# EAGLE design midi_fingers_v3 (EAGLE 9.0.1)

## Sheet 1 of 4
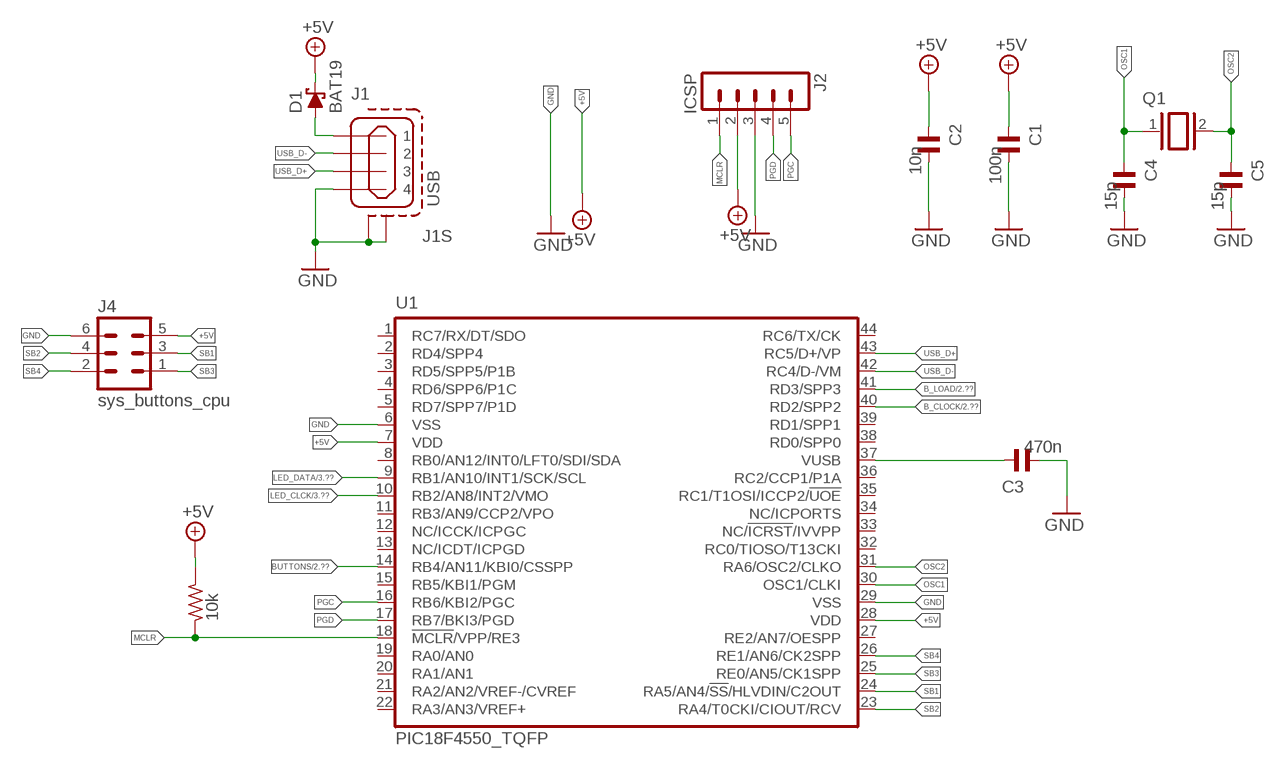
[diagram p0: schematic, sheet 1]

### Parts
C1  100n  C-EUC0603  [C0603]
C2  10n  C-EUC0603  [C0603]
C3  470n  C-EUC0603K  [C0603K]
C4  15p  C-EUC0603  [C0603]
C5  15p  C-EUC0603  [C0603]
D1  BAT19  [DO35-10]
J1  USB  MINI-USB_SHIELD4P-85-32004-00X  [85-32004-00X]
J2  ICSP  MA05-1  [MA05-1]
J4  sys_buttons_cpu  MA03-2  [MA03-2]
Q1  XTAL/S  [QS]
R2  10k  R-EU_M2012  [M2012]
U1  PIC18F4550_TQFP  [TQFP44]

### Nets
+5V: C1.2 C2.2 D1.C J2.2 J4.5 R2.1 U1.7(VDD) U1.28(VDD) ; also sheet 2,3,4
+5V__: D1.A J1.1
B_CLOCK: U1.40(RD2/SPP2) ; also sheet 2
B_LOAD: U1.41(RD3/SPP3) ; also sheet 2
BUTTONS: U1.14(RB4/AN11/KBI0/CSSPP) ; also sheet 2
GND: C1.1 C2.1 C3.1 C4.1 C5.1 J1.4 J1.M1(S1) J1.M2(S2) J2.3 J4.6 U1.6(VSS) U1.29(VSS) ; also sheet 2,3,4
LED_CLCK: U1.10(RB2/AN8/INT2/VMO) ; also sheet 3
LED_DATA: U1.9(RB1/AN10/INT1/SCK/SCL) ; also sheet 3
MCLR: J2.1 R2.2 U1.18(!MCLR!/VPP/RE3)
N$5: C3.2 U1.37(VUSB)
OSC1: C4.2 Q1.1 U1.30(OSC1/CLKI)
OSC2: C5.2 Q1.2 U1.31(RA6/OSC2/CLKO)
PGC: J2.5 U1.16(RB6/KBI2/PGC)
PGD: J2.4 U1.17(RB7/BKI3/PGD)
SB1: J4.3 U1.24(RA5/AN4/!SS!/HLVDIN/C2OUT)
SB2: J4.4 U1.23(RA4/T0CKI/CIOUT/RCV)
SB3: J4.1 U1.25(RE0/AN5/CK1SPP)
SB4: J4.2 U1.26(RE1/AN6/CK2SPP)
USB_D+: J1.3 U1.43(RC5/D+/VP)
USB_D-: J1.2 U1.42(RC4/D-/VM)
Unconnected: U1.1(RC7/RX/DT/SDO) U1.2(RD4/SPP4) U1.3(RD5/SPP5/P1B) U1.4(RD6/SPP6/P1C) U1.5(RD7/SPP7/P1D) U1.8(RB0/AN12/INT0/LFT0/SDI/SDA) U1.11(RB3/AN9/CCP2/VPO) U1.12(NC/ICCK/ICPGC) U1.13(NC/ICDT/ICPGD) U1.15(RB5/KBI1/PGM) U1.19(RA0/AN0) U1.20(RA1/AN1) U1.21(RA2/AN2/VREF-/CVREF) U1.22(RA3/AN3/VREF+) U1.27(RE2/AN7/OESPP) U1.32(RC0/TIOSO/T13CKI) U1.33(NC/!ICRST!/IVVPP) U1.34(NC/ICPORTS) U1.35(RC1/T1OSI/ICCP2/!UOE) U1.36(RC2/CCP1/P1A) U1.38(RD0/SPP0) U1.39(RD1/SPP1) U1.44(RC6/TX/CK)

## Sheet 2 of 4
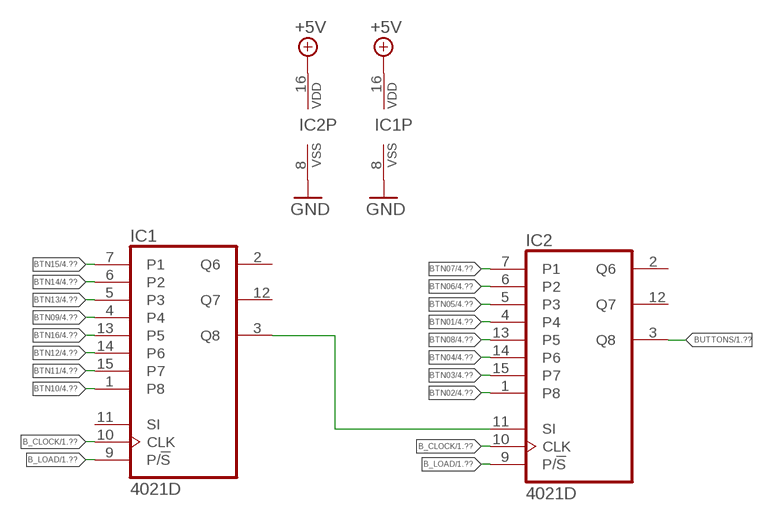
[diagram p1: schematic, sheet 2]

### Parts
IC1  4021D  [SO16]
IC2  4021D  [SO16]

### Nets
+5V: IC1.16(VDD) IC2.16(VDD) ; also sheet 1,3,4
B_CLOCK: IC1.10(CLK) IC2.10(CLK) ; also sheet 1
B_LOAD: IC1.9(P/!S) IC2.9(P/!S) ; also sheet 1
BTN01: IC2.4 ; also sheet 4
BTN02: IC2.1(P8) ; also sheet 4
BTN03: IC2.15(P7) ; also sheet 4
BTN04: IC2.14(P6) ; also sheet 4
BTN05: IC2.5(P3) ; also sheet 4
BTN06: IC2.6(P2) ; also sheet 4
BTN07: IC2.7(P1) ; also sheet 4
BTN08: IC2.13(P5) ; also sheet 4
BTN09: IC1.4 ; also sheet 4
BTN10: IC1.1(P8) ; also sheet 4
BTN11: IC1.15(P7) ; also sheet 4
BTN12: IC1.14(P6) ; also sheet 4
BTN13: IC1.5(P3) ; also sheet 4
BTN14: IC1.6(P2) ; also sheet 4
BTN15: IC1.7(P1) ; also sheet 4
BTN16: IC1.13(P5) ; also sheet 4
BTN_SERIAL: IC1.3(Q8) IC2.11(SI)
BUTTONS: IC2.3(Q8) ; also sheet 1
GND: IC1.8(VSS) IC2.8(VSS) ; also sheet 1,3,4
Unconnected: IC1.2(Q6) IC1.11(SI) IC1.12(Q7) IC2.2(Q6) IC2.12(Q7)

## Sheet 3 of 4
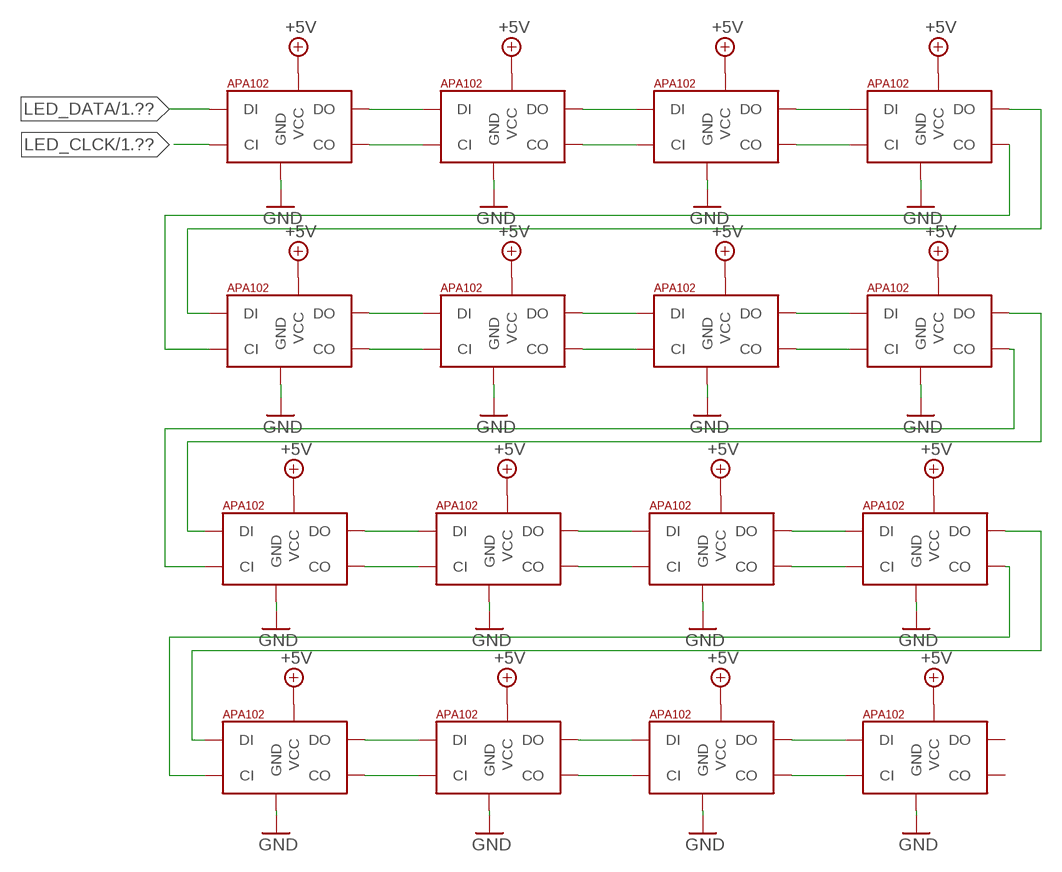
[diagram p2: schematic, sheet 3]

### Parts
LED1  APA1025050  [APA102_5050]
LED2  APA1025050  [APA102_5050]
LED3  APA1025050  [APA102_5050]
LED4  APA1025050  [APA102_5050]
LED5  APA1025050  [APA102_5050]
LED6  APA1025050  [APA102_5050]
LED7  APA1025050  [APA102_5050]
LED8  APA1025050  [APA102_5050]
LED9  APA1025050  [APA102_5050]
LED10  APA1025050  [APA102_5050]
LED11  APA1025050  [APA102_5050]
LED12  APA1025050  [APA102_5050]
LED13  APA1025050  [APA102_5050]
LED14  APA1025050  [APA102_5050]
LED15  APA1025050  [APA102_5050]
LED16  APA1025050  [APA102_5050]

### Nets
+5V: LED1.1(VCC) LED2.1(VCC) LED3.1(VCC) LED4.1(VCC) LED5.1(VCC) LED6.1(VCC) LED7.1(VCC) LED8.1(VCC) LED9.1(VCC) LED10.1(VCC) LED11.1(VCC) LED12.1(VCC) LED13.1(VCC) LED14.1(VCC) LED15.1(VCC) LED16.1(VCC) ; also sheet 1,2,4
GND: LED1.6(GND) LED2.6(GND) LED3.6(GND) LED4.6(GND) LED5.6(GND) LED6.6(GND) LED7.6(GND) LED8.6(GND) LED9.6(GND) LED10.6(GND) LED11.6(GND) LED12.6(GND) LED13.6(GND) LED14.6(GND) LED15.6(GND) LED16.6(GND) ; also sheet 1,2,4
LED_CLCK: LED1.5(CI) ; also sheet 1
LED_DATA: LED1.4(DI) ; also sheet 1
N$1: LED1.3(DO) LED2.4(DI)
N$2: LED2.3(DO) LED3.4(DI)
N$3: LED3.3(DO) LED4.4(DI)
N$4: LED5.3(DO) LED6.4(DI)
N$6: LED6.3(DO) LED7.4(DI)
N$7: LED7.3(DO) LED8.4(DI)
N$8: LED9.3(DO) LED10.4(DI)
N$9: LED10.3(DO) LED11.4(DI)
N$10: LED11.3(DO) LED12.4(DI)
N$11: LED13.3(DO) LED14.4(DI)
N$12: LED14.3(DO) LED15.4(DI)
N$13: LED15.3(DO) LED16.4(DI)
N$14: LED8.3(DO) LED9.4(DI)
N$15: LED12.3(DO) LED13.4(DI)
N$16: LED1.2(CO) LED2.5(CI)
N$17: LED2.2(CO) LED3.5(CI)
N$18: LED3.2(CO) LED4.5(CI)
N$19: LED4.3(DO) LED5.4(DI)
N$20: LED4.2(CO) LED5.5(CI)
N$21: LED5.2(CO) LED6.5(CI)
N$22: LED6.2(CO) LED7.5(CI)
N$23: LED7.2(CO) LED8.5(CI)
N$24: LED8.2(CO) LED9.5(CI)
N$25: LED9.2(CO) LED10.5(CI)
N$26: LED10.2(CO) LED11.5(CI)
N$27: LED11.2(CO) LED12.5(CI)
N$28: LED12.2(CO) LED13.5(CI)
N$30: LED13.2(CO) LED14.5(CI)
N$31: LED14.2(CO) LED15.5(CI)
N$32: LED15.2(CO) LED16.5(CI)
Unconnected: LED16.2(CO) LED16.3(DO)

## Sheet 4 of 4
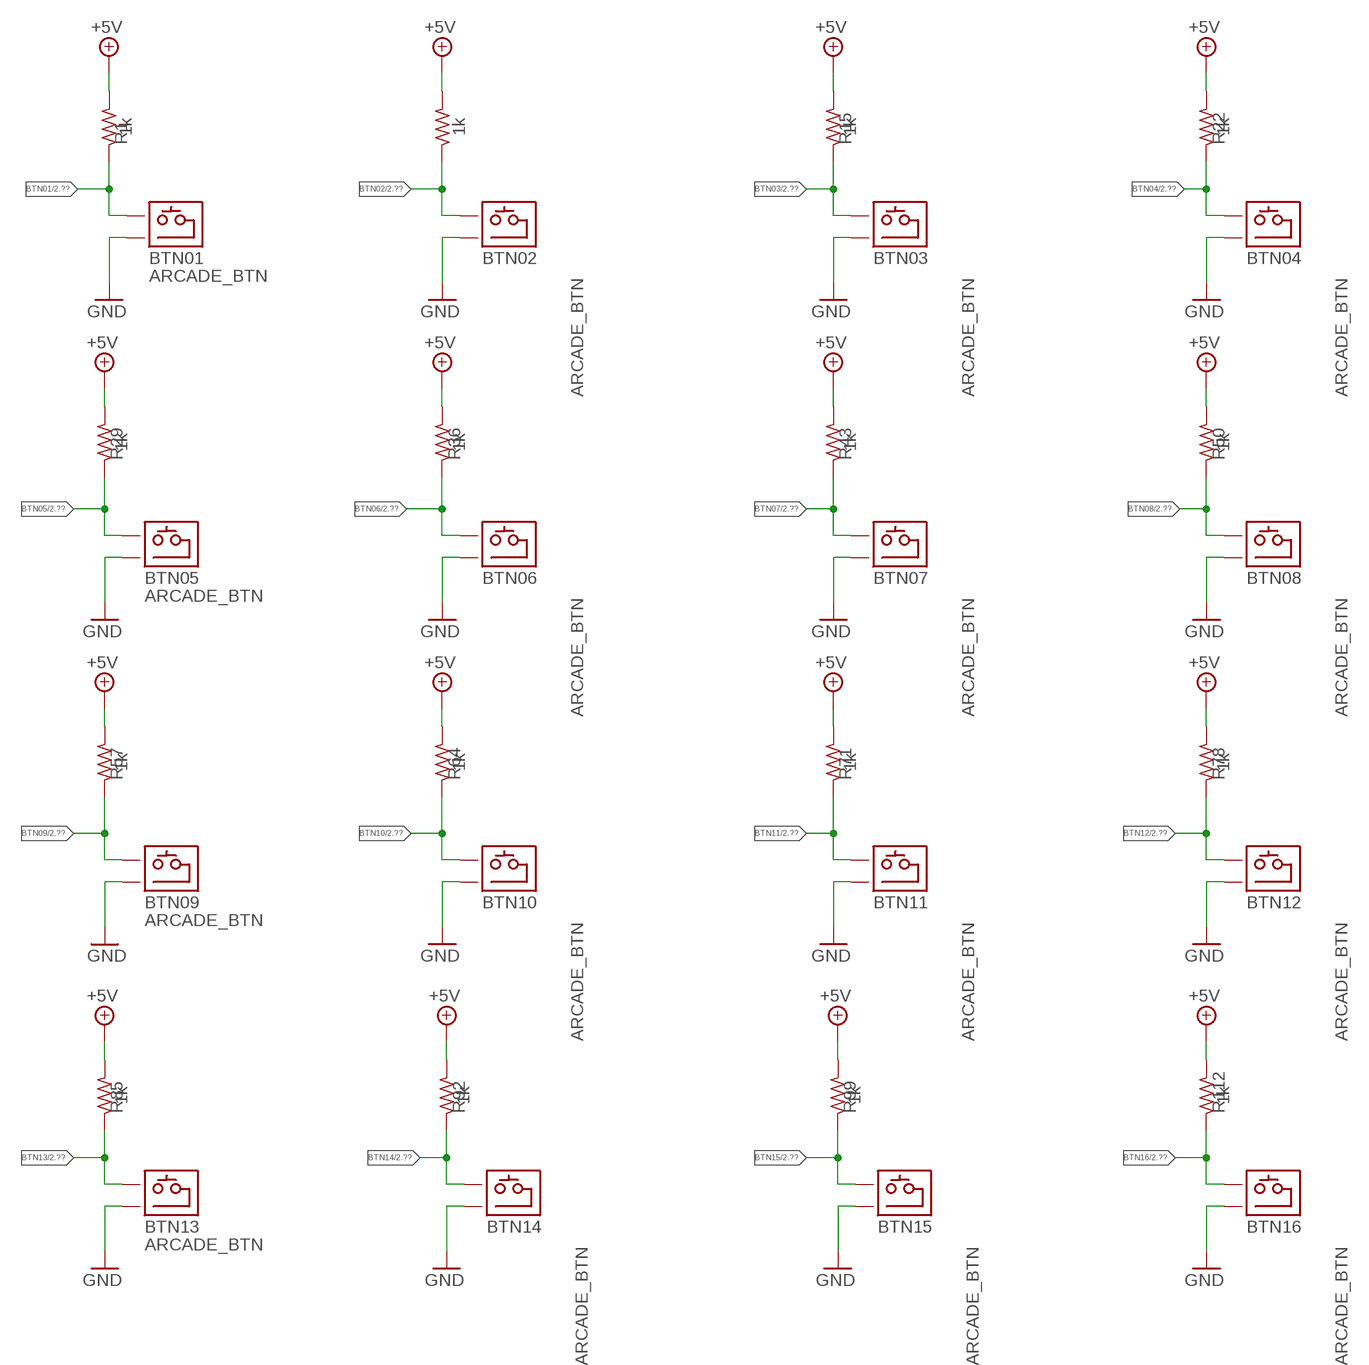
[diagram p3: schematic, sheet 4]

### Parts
BTN01  ARCADE_BTN  [ARCADE_BTN_ALONE]
BTN02  ARCADE_BTN  [ARCADE_BTN_ALONE]
BTN03  ARCADE_BTN  [ARCADE_BTN_ALONE]
BTN04  ARCADE_BTN  [ARCADE_BTN_ALONE]
BTN05  ARCADE_BTN  [ARCADE_BTN_ALONE]
BTN06  ARCADE_BTN  [ARCADE_BTN_ALONE]
BTN07  ARCADE_BTN  [ARCADE_BTN_ALONE]
BTN08  ARCADE_BTN  [ARCADE_BTN_ALONE]
BTN09  ARCADE_BTN  [ARCADE_BTN_ALONE]
BTN10  ARCADE_BTN  [ARCADE_BTN_ALONE]
BTN11  ARCADE_BTN  [ARCADE_BTN_ALONE]
BTN12  ARCADE_BTN  [ARCADE_BTN_ALONE]
BTN13  ARCADE_BTN  [ARCADE_BTN_ALONE]
BTN14  ARCADE_BTN  [ARCADE_BTN_ALONE]
BTN15  ARCADE_BTN  [ARCADE_BTN_ALONE]
BTN16  ARCADE_BTN  [ARCADE_BTN_ALONE]
R1  1k  R-EU_M2012  [M2012]
R8  1k  R-EU_M2012  [M2012]
R15  1k  R-EU_M2012  [M2012]
R22  1k  R-EU_M2012  [M2012]
R29  1k  R-EU_M2012  [M2012]
R36  1k  R-EU_M2012  [M2012]
R43  1k  R-EU_M2012  [M2012]
R50  1k  R-EU_M2012  [M2012]
R57  1k  R-EU_M2012  [M2012]
R64  1k  R-EU_M2012  [M2012]
R71  1k  R-EU_M2012  [M2012]
R78  1k  R-EU_M2012  [M2012]
R85  1k  R-EU_M2012  [M2012]
R92  1k  R-EU_M2012  [M2012]
R99  1k  R-EU_M2012  [M2012]
R112  1k  R-EU_M2012  [M2012]

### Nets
+5V: R1.1 R8.1 R15.1 R22.1 R29.1 R36.1 R43.1 R50.1 R57.1 R64.1 R71.1 R78.1 R85.1 R92.1 R99.1 R112.1 ; also sheet 1,2,3
BTN01: BTN01.1(B1) R1.2 ; also sheet 2
BTN02: BTN02.1(B1) R8.2 ; also sheet 2
BTN03: BTN03.1(B1) R15.2 ; also sheet 2
BTN04: BTN04.1(B1) R22.2 ; also sheet 2
BTN05: BTN05.1(B1) R29.2 ; also sheet 2
BTN06: BTN06.1(B1) R36.2 ; also sheet 2
BTN07: BTN07.1(B1) R43.2 ; also sheet 2
BTN08: BTN08.1(B1) R50.2 ; also sheet 2
BTN09: BTN09.1(B1) R57.2 ; also sheet 2
BTN10: BTN10.1(B1) R64.2 ; also sheet 2
BTN11: BTN11.1(B1) R71.2 ; also sheet 2
BTN12: BTN12.1(B1) R78.2 ; also sheet 2
BTN13: BTN13.1(B1) R85.2 ; also sheet 2
BTN14: BTN14.1(B1) R92.2 ; also sheet 2
BTN15: BTN15.1(B1) R99.2 ; also sheet 2
BTN16: BTN16.1(B1) R112.2 ; also sheet 2
GND: BTN01.2(B2) BTN02.2(B2) BTN03.2(B2) BTN04.2(B2) BTN05.2(B2) BTN06.2(B2) BTN07.2(B2) BTN08.2(B2) BTN09.2(B2) BTN10.2(B2) BTN11.2(B2) BTN12.2(B2) BTN13.2(B2) BTN14.2(B2) BTN15.2(B2) BTN16.2(B2) ; also sheet 1,2,3

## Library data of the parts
BTN01-BTN09 BTN10-BTN16 = arcade-button:ARCADE_BTN
C1-C5 = rcl:C-EU: CAPACITOR, European symbol
D1 = diode:BAT19: DIODE
IC1 IC2 = 40xx:4021: 8-bit static SHIFT REGISTER
J1 = con-cypressindustries:MINI-USB_SHIELD4P-: MINI USB 4 Pol. Source: www.cypressindustries.com
J2 = con-lstb:MA05-1: PIN HEADER; OC_FARNELL: unknown; OC_NEWARK: unknown
J4 = con-lstb:MA03-2: PIN HEADER
LED1-LED16 = jos-ph:APA102: APA102C 5050 RGB LED -- Adafruit DotStar Single LED Pixel Product Page: https://www.adafruit.com/products/2343 Datasheet: https://cdn-shop.adafruit.com/product-files/2343/APA102C.pdf
Q1 = special:XTAL/S: CRYSTAL
R1 R2 R8 R15 R22 R29 R36 R43 R50 R57 R64 R71 R78 R85 R92 R99 R112 = rcl:R-EU_: RESISTOR, European symbol
U1 = microchip:PIC18F4*_TQFP: USB Microcontrollers with nanoWatt Technology High-Performance, Enhanced Flash, 28/40/44-Pin, Source: http://ww1.microchip.com/downloads/en/devicedoc/39632c.pdf

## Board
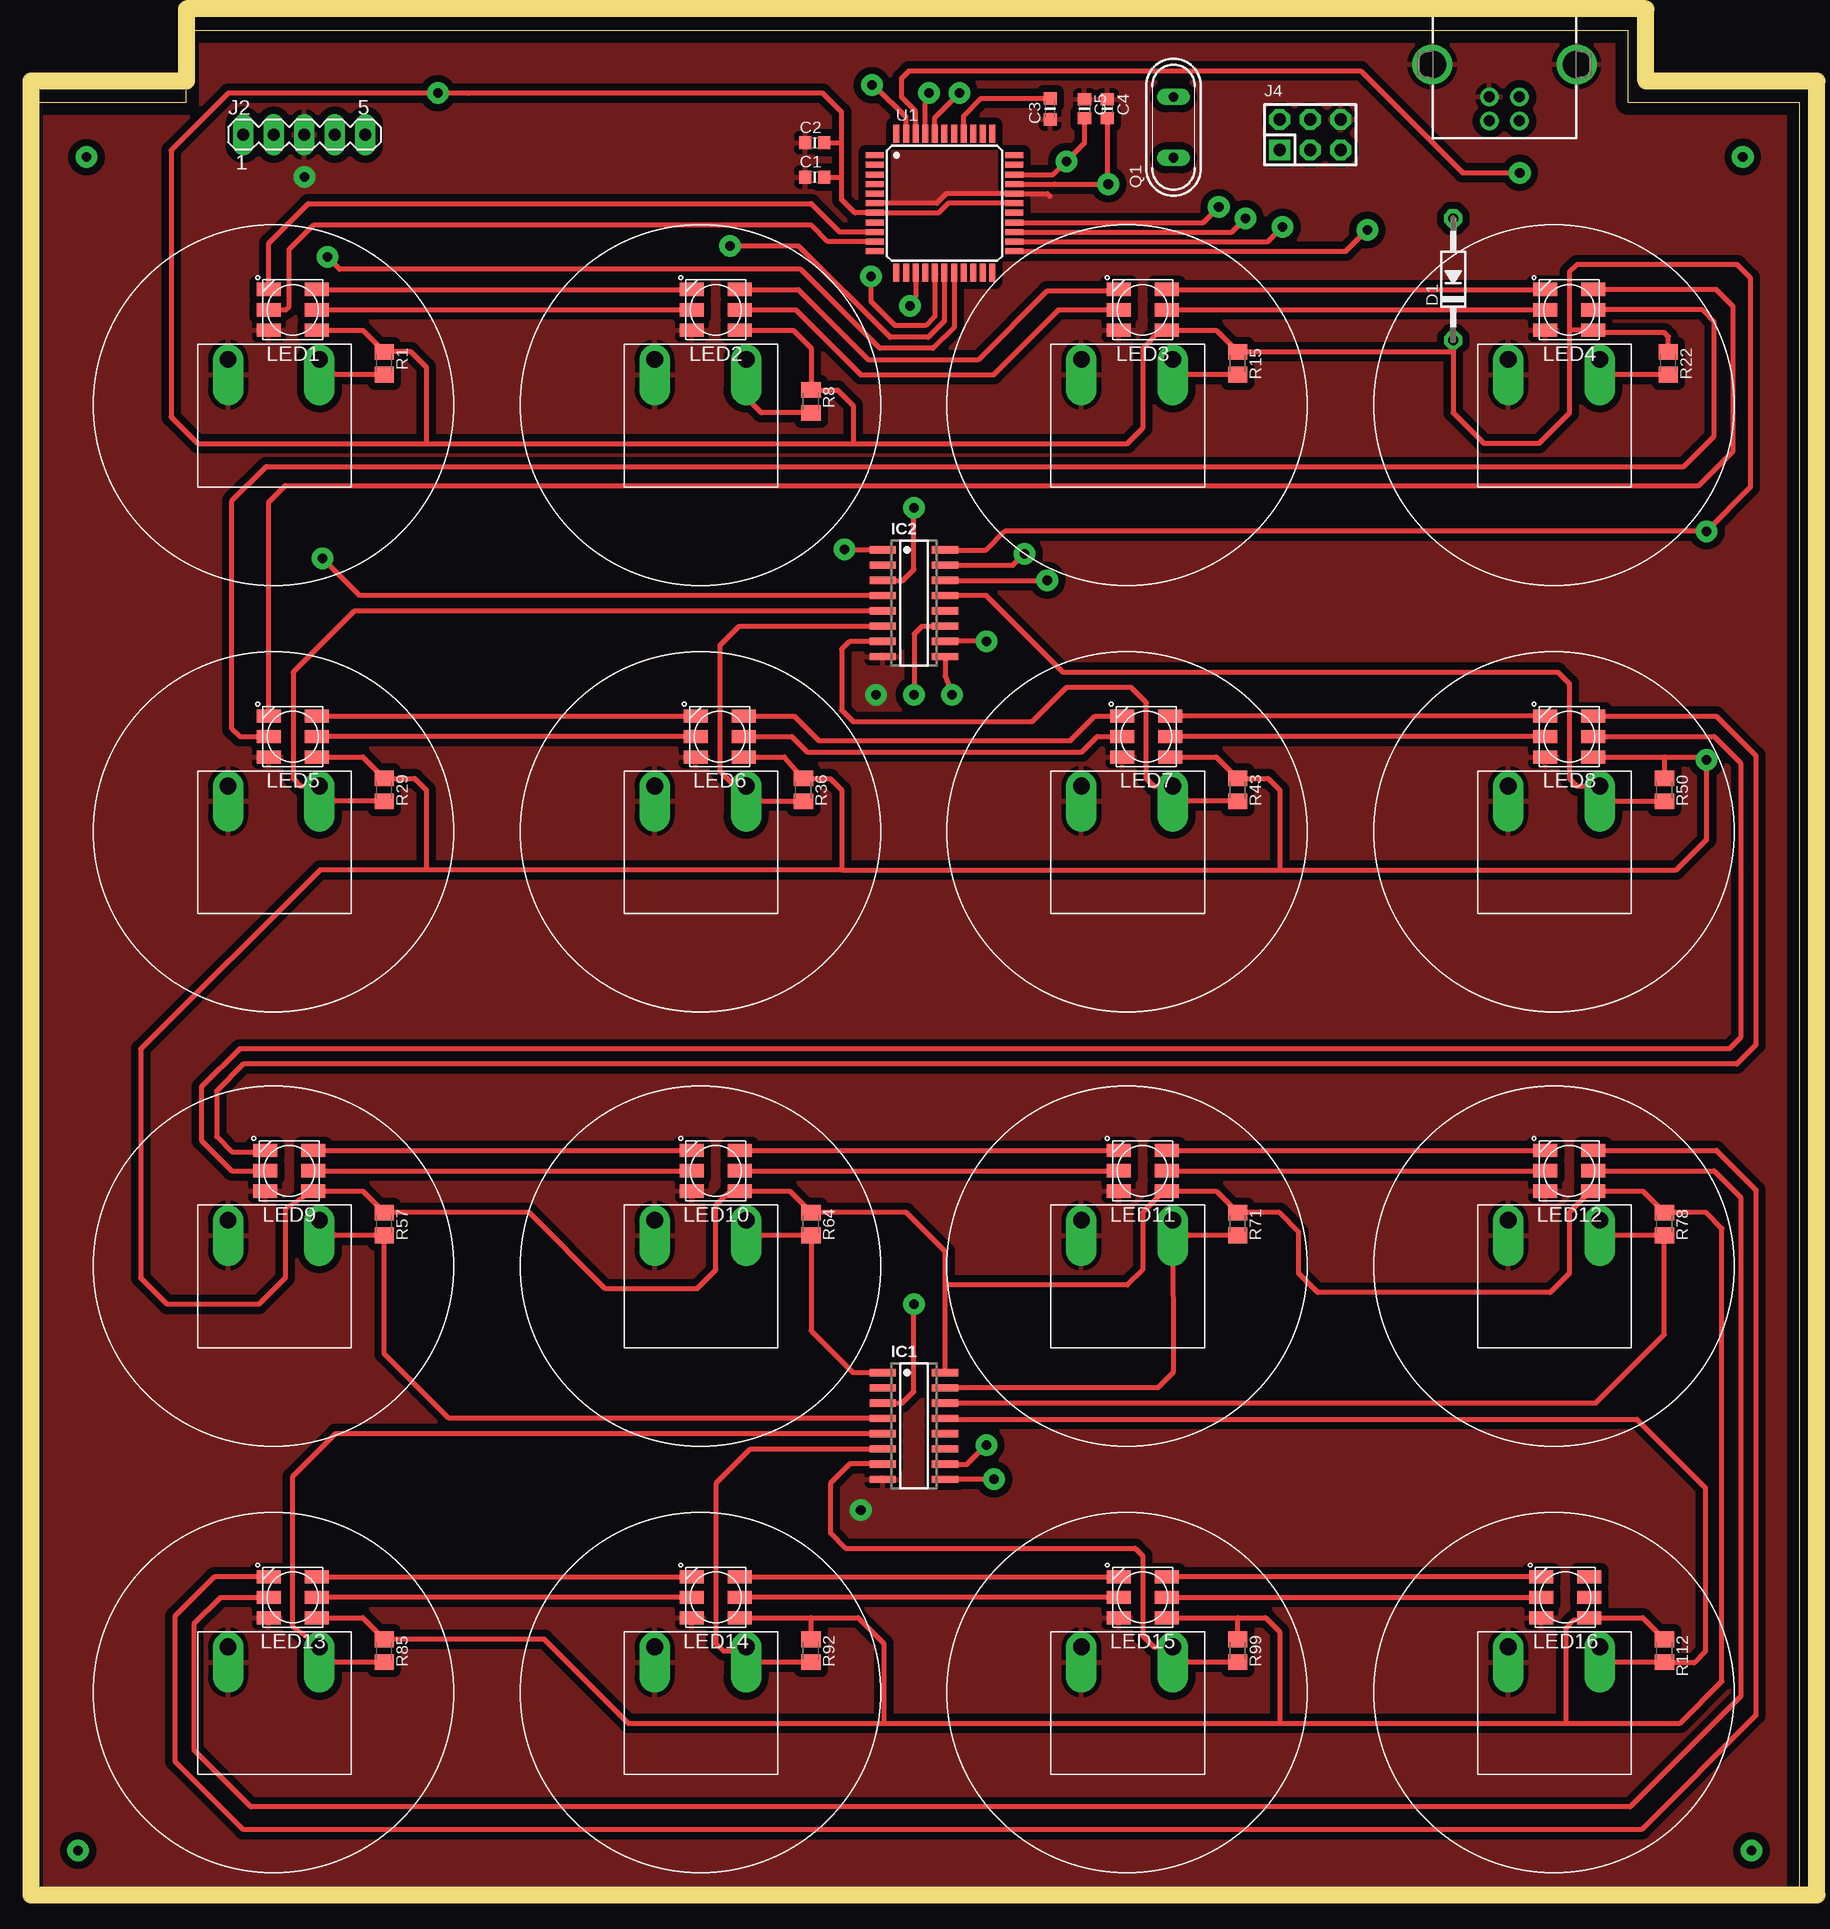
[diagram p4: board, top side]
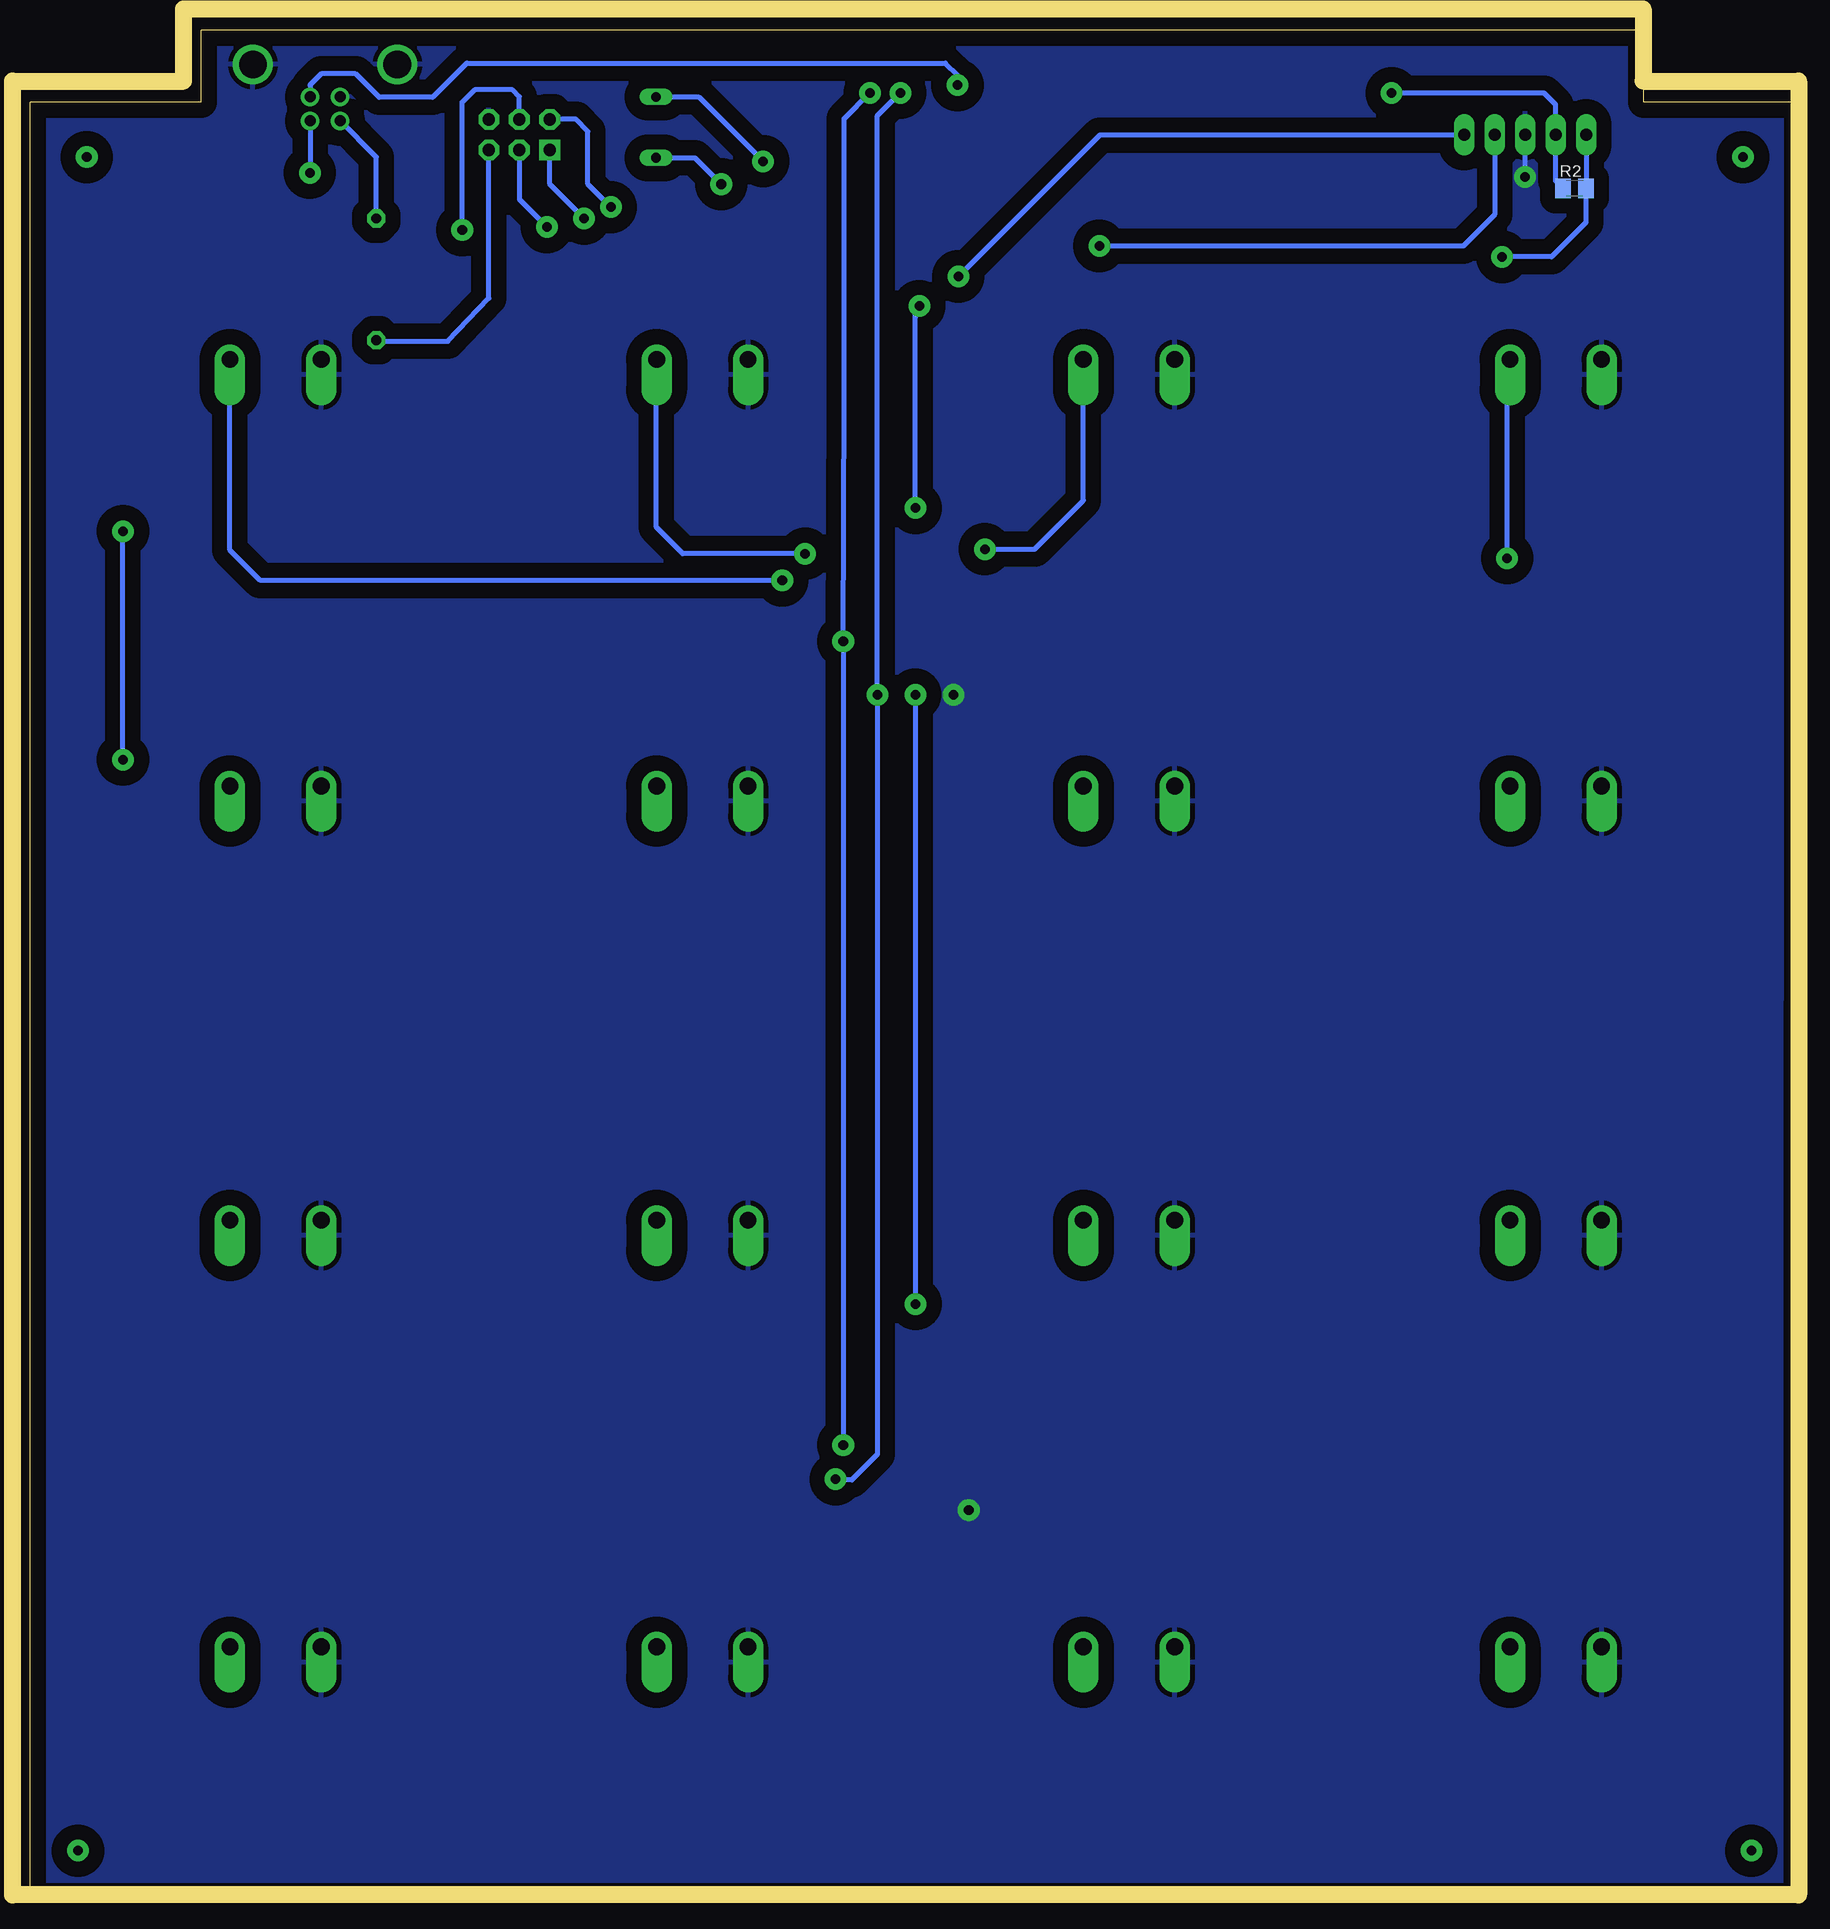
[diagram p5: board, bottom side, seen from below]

Size 147.46 x 155.76 mm. Coordinates in mm from the lower left corner, seen from the top.
Outline: 0.01,0 147.46,0 147.46,149.76 133.19,149.76 133.19,155.76 13,155.76 13,149.76 0,149.76 0.01,0
Copper layers (1*16): Top 0.035mm / dielectric 1.5mm / Bottom 0.035mm
Design rules "default *": minimum track width 10mil, minimum drill 0.6mm, track to track 8mil, track to pad 8mil, pad to pad 8mil, via to via 8mil, smd to smd 8mil, copper to edge 40mil, drill to drill 6mil, minimum pad ring 0mil, minimum via ring 8mil, stop-mask expansion 4mil, vias tented up to drill 0mil, thermal gap 16mil
Milling: 8 lines

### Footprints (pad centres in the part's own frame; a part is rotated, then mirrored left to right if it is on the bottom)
ARCADE_BTN_ALONE = drill 1.4 pad 2.54 offset: 1 3.81,3.81; 2 -3.81,3.81
C0603 = smd 1 x 1.1: 1 -0.794,0; 2 0.794,0
C0603K = smd 1.05 x 1.08: 1 -0.875,0; 2 0.875,0
DO35-10 = drill 0.813 pad 1.524 octagon: A 5.08,0; C -5.08,0
SO16 = smd 0.6 x 2.2: 1 -4.445,-2.6; 2 -3.175,-2.6; 3 -1.905,-2.6; 4 -0.635,-2.6; 5 0.635,-2.6; 6 1.905,-2.6; 7 3.175,-2.6; 8 4.445,-2.6; 9 4.445,2.6; 10 3.175,2.6; 11 1.905,2.6; 12 0.635,2.6; 13 -0.635,2.6; 14 -1.905,2.6; 15 -3.175,2.6; 16 -4.445,2.6
85-32004-00X = drill 0.92 pad 1.27: 1 4.71,-1.25; 2 4.71,1.25; 3 2.71,1.25; 4 2.71,-1.25 | drill 2.3 pad 3: M1 0,6.02; M2 0,-6.02
MA05-1 = drill 1.016 long: 1 -5.08,0; 2 -2.54,0; 3 0,0; 4 2.54,0; 5 5.08,0
MA03-2 = drill 1.016 square: 1 -2.54,-1.27 | drill 1.016 octagon: 2 -2.54,1.27; 3 0,-1.27; 4 0,1.27; 5 2.54,-1.27; 6 2.54,1.27
APA102_5050 = smd 2 x 1.1: 1 2,-1.7; 2 2,0; 3 2,1.7; 4 -2,1.7; 5 -2,0; 6 -2,-1.7
QS = drill 0.8 long: 1 -2.54,0; 2 2.54,0
M2012 = smd 1.3 x 1.6: 1 -0.95,0; 2 0.95,0
TQFP44 = smd 1.5 x 0.5: 1 -5.8,4; 2 -5.8,3.2; 3 -5.8,2.4; 4 -5.8,1.6; 5 -5.8,0.8; 6 -5.8,0; 7 -5.8,-0.8; 8 -5.8,-1.6; 9 -5.8,-2.4; 10 -5.8,-3.2; 11 -5.8,-4; 23 5.8,-4; 24 5.8,-3.2; 25 5.8,-2.4; 26 5.8,-1.6; 27 5.8,-0.8; 28 5.8,0; 29 5.8,0.8; 30 5.8,1.6; 31 5.8,2.4; 32 5.8,3.2; 33 5.8,4 | smd 0.5 x 1.5: 12 -4,-5.8; 13 -3.2,-5.8; 14 -2.4,-5.8; 15 -1.6,-5.8; 16 -0.8,-5.8; 17 0,-5.8; 18 0.8,-5.8; 19 1.6,-5.8; 20 2.4,-5.8; 21 3.2,-5.8; 22 4,-5.8; 34 4,5.8; 35 3.2,5.8; 36 2.4,5.8; 37 1.6,5.8; 38 0.8,5.8; 39 0,5.8; 40 -0.8,5.8; 41 -1.6,5.8; 42 -2.4,5.8; 43 -3.2,5.8; 44 -4,5.8

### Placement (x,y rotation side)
BTN01  20.31,124.49 0 top
BTN02  55.87,124.49 0 top
BTN03  91.43,124.49 0 top
BTN04  126.99,124.49 0 top
BTN05  20.31,88.93 0 top
BTN06  55.87,88.93 0 top
BTN07  91.43,88.93 0 top
BTN08  126.99,88.93 0 top
BTN09  20.31,52.73 0 top
BTN10  55.87,52.73 0 top
BTN11  91.43,52.73 0 top
BTN12  126.99,52.73 0 top
BTN13  20.31,17.17 0 top
BTN14  55.87,17.17 0 top
BTN15  91.43,17.17 0 top
BTN16  126.99,17.17 0 top
C1  65.39,143.5 0 top
C2  65.39,146.35 0 top
C3  85.01,149.19 90 top
C4  89.78,149.19 270 top
C5  87.87,149.19 270 top
D1  118.6,134.97 90 top
IC1  73.66,39.4 270 top
IC2  73.66,107.98 270 top
J1  122.87,152.89 270 top
J2  22.86,147.03 0 top
J4  106.68,147.03 0 top
LED1  21.91,132.43 0 top
LED2  57.15,132.43 0 top
LED3  92.71,132.43 0 top
LED4  128.27,132.43 0 top
LED5  21.91,96.86 0 top
LED6  57.47,96.86 0 top
LED7  93.03,96.86 0 top
LED8  128.27,96.86 0 top
LED9  21.59,60.67 0 top
LED10  57.15,60.67 0 top
LED11  92.71,60.67 0 top
LED12  128.27,60.67 0 top
LED13  21.91,25.11 0 top
LED14  57.15,25.11 0 top
LED15  92.71,25.11 0 top
LED16  127.95,25.11 0 top
Q1  95.29,147.65 90 top
R1  29.53,127.98 270 top
R2  18.75,142.56 0 bottom
R8  65.09,124.81 270 top
R15  100.65,127.98 270 top
R22  136.52,127.98 270 top
R29  29.53,92.42 270 top
R36  64.45,92.42 270 top
R43  100.65,92.42 270 top
R50  136.21,92.42 270 top
R57  29.53,56.23 270 top
R64  65.09,56.23 270 top
R71  100.65,56.23 270 top
R78  136.21,56.23 270 top
R85  29.53,20.66 270 top
R92  65.09,20.66 270 top
R99  100.65,20.66 270 top
R112  136.21,20.66 270 top
U1  76.2,141.31 0 top

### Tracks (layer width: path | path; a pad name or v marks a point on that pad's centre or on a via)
+5V  (via drill 0.8 pad 1.8)
  Top 0.406: R22.1 136.52,130.2 136.21,130.52 130.48,130.52 LED4.1 | R15.1 | R15.1 98.85,130.72 LED3.1 94.18,130.72 92.71,129.25 92.71,122.57 92.72,122.56 91.45,121.28 68.59,121.28 | LED1.1 27.73,130.72 R1.1 | LED5.1 27.73,95.17 R29.1 32.05,93.37 33.03,92.39 33.03,85.75 | LED6.1 62.86,95.17 R36.1 64.48,93.34 66.69,93.34 67.64,92.39 67.64,85.75 | 76.26,51.4 IC1.16 76.33,43.77 | 76.26,51.4 76.26,53.94 73.03,57.18 R64.1 63.29,58.97 LED10.1 | LED10.1 59.15,58.86 | 100.65,23.41 LED15.1 94.17,23.41 | R99.1 100.65,23.41 | LED13.1 27.73,23.41 R85.1 42.86,21.62 49.85,14.63 71.13,14.63 | LED16.1 134.41,23.41 R112.1 | LED16.1 129.74,23.41 | R1.1 | LED7.1 94.82,95.17 | U1.28 76.52,141.31 75.72,140.51 U1.7 68.73,140.51 67.64,141.6 67.64,143.51 | LED14.1 65.09,23.41 | 65.09,23.41 69.01,23.41 71.13,21.29 71.13,14.63 | R92.1 65.09,23.41 | 76.26,51.4 76.51,51.15 91.44,51.15 92.71,52.41 92.71,57.18 94.5,58.97 LED11.1 98.85,58.97 R71.1 104.14,57.18 105.73,55.59 105.73,52.1 107.31,50.51 126.68,50.51 128.27,52.1 128.27,57.18 129.95,58.86 LED12.1 134.41,58.97 R78.1 139.69,57.17 140.98,55.88 140.98,18.1 137.52,14.63 127.97,14.63 | IC2.16 79.68,112.42 81.24,113.98 v139.71,113.98 143.36,117.63 143.36,135.1 142.25,136.21 128.92,136.21 128.28,135.57 128.28,130.81 | 129.73,130.72 LED4.1 | R15.1 118.59,128.93 D1.C 118.6,123.85 121.17,121.28 125.74,121.28 128.28,123.83 128.28,130.81 | LED16.1 129.91,23.45 | LED4.1 128.37,130.72 128.28,130.81 | LED7.1 94.94,95.25 | LED10.1 58.11,58.74 57.16,57.78 57.15,52.41 55.56,50.83 47.94,50.83 41.59,57.18 R57.1 27.73,58.97 LED9.1 21.29,57.47 21.29,51.75 19.06,49.53 11.44,49.53 9.22,51.75 9.22,70.8 24.17,85.75 33.03,85.75
  Top 0.406: LED16.1 129.72,23.18 128.6,23.18 127.97,22.54 127.97,14.63 | 71.13,14.63 104.15,14.63 | 104.15,14.63 127.97,14.63 | 100.65,23.41 102.97,23.41 104.15,22.23 104.15,14.63 | LED8.1 136.22,95.17 | 136.22,95.17 139.48,95.17 v139.71,94.93 139.71,88.27 137.2,85.75 104.15,85.75 | R50.1 136.22,93.38 136.22,95.17 | R43.1 100.66,93.38 | 67.64,85.75 104.15,85.75 | 67.64,143.51 67.64,147 | 67.64,147 67.64,148.91 66.05,150.5 36.53,150.5 | R1.1 31.74,128.93 33.03,127.64 33.03,121.28 | 36.53,150.5 v33.98,150.5 33.67,150.5 | 33.67,150.5 16.52,150.5 11.76,145.73 11.76,123.51 13.98,121.28 33.03,121.28 | J2.2 20.33,147.04 | 58.67,130.72 LED2.1 63.61,130.72 65.09,129.25 R8.1 67.3,125.75 68.59,124.46 68.59,121.28 | 67.64,85.75 33.03,85.75 | LED7.1 98.85,95.17 R43.1 | R43.1 103.17,93.37 104.15,92.39 104.15,85.75 | 33.03,121.28 68.59,121.28 | 33.68,150.48 33.67,150.5 | 36.54,150.48 36.53,150.5 | C2.2 67.63,146.35 67.64,147 | C1.2 67.63,143.5 67.64,143.51
  Bottom 0.406: D1.C 118.52,129.82 112.64,129.82 109.22,133.39 J4.5 | v139.71,94.93 v139.71,113.98 | v33.98,150.5 21.29,150.5 20.32,149.53 J2.2 20.32,143.18 R2.1
+5V__
  Bottom 0.406: D1.A 118.6,145.16 J1.1
B_CLOCK  (via drill 0.8 pad 1.8)
  Top 0.406: U1.40 75.4,148.45 v77.47,150.52 | v79.69,37.81 78.04,36.16 76.44,36.16 IC1.10 | v79.69,104.8 IC2.10
  Bottom 0.406: v79.69,37.81 v79.69,104.8 79.62,125.06 79.62,148.38 v77.47,150.52
B_LOAD  (via drill 0.8 pad 1.8)
  Top 0.406: IC2.9 76.26,101.89 v76.84,100.36 | v80.33,34.95 IC1.9 | U1.41 74.6,150.19 v74.93,150.52
  Bottom 0.406: v80.33,34.95 80.26,34.88 78.98,34.88 76.84,37.03 v76.84,100.36 76.84,148.62 v74.93,150.52
BTN01  (via drill 0.8 pad 1.8)
  Top 0.406: IC2.4 27.48,108.61 v24.37,111.72 | R1.2 25.39,127.03 BTN01.1
  Bottom 0.406: v24.37,111.72 24.37,128.05 BTN01.1
BTN02  (via drill 0.8 pad 1.8)
  Top 0.406: R8.2 60.94,123.86 59.68,125.12 BTN02.1 | IC2.1 67.95,112.42 v67.89,112.48
  Bottom 0.406: v67.89,112.48 63.74,112.48 59.68,116.55 BTN02.1
BTN03  (via drill 0.8 pad 1.8)
  Top 0.406: R15.2 96.52,127.03 BTN03.1 | v82.87,112.11 81.92,111.15 IC2.15
  Bottom 0.406: v82.87,112.11 93.07,112.11 95.26,114.3 95.26,128.28 BTN03.1
BTN04  (via drill 0.8 pad 1.8)
  Top 0.406: IC2.14 v84.77,109.88 | R22.2 132.07,127.03 BTN04.1
  Bottom 0.406: v84.77,109.88 128.27,109.88 130.8,112.41 BTN04.1
BTN05
  Top 0.406: R29.2 25.4,91.47 BTN05.1 22.58,92.74 22.56,92.71 21.92,93.34 21.92,102.23 27,107.31 71.03,107.31 IC2.5
BTN06
  Top 0.406: 65.09,91.47 R36.2 60.95,91.47 BTN06.1 58.72,92.74 57.48,93.98 57.48,104.46 59.07,106.05 71.03,106.05 IC2.6
BTN07
  Top 0.406: R43.2 96.52,91.47 BTN07.1 95.21,92.71 93.67,92.71 93.04,93.34 93.04,99.69 91.77,100.97 86.37,100.97 83.51,98.11 68.59,98.11 67.64,99.06 67.64,104.14 68.28,104.78 71.03,104.78 IC2.7
BTN08
  Top 0.406: IC2.13 79.69,108.61 86.07,102.23 127.33,102.23 128.28,101.28 128.28,93.34 128.89,92.74 BTN08.1 132.07,91.47 R50.2
BTN09
  Top 0.406: R57.2 | R57.2 | R57.2 29.22,55.27 | 29.22,55.27 25.4,55.27 BTN09.1 | 29.22,55.27 29.54,54.96 29.54,45.4 34.91,40.03 IC1.4
BTN10
  Top 0.406: R64.2 | R64.2 65.09,47.34 68.58,43.84 IC1.1 | R64.2 60.96,55.27 BTN10.1
BTN11
  Top 0.406: IC1.15 93.98,42.57 95.25,43.84 BTN11.1 96.52,55.27 R71.2
BTN12
  Top 0.406: R78.2 | IC1.14 130.49,41.3 136.21,47.02 R78.2 | R78.2 132.08,55.27 BTN12.1
BTN13
  Top 0.406: R85.2 25.4,19.71 BTN13.1 24.12,21.07 21.87,22.69 21.87,35.15 25.48,38.76 IC1.5
BTN14
  Top 0.406: R92.2 60.96,19.71 60.02,20.64 | IC1.6 70.99,37.42 59.98,37.42 57.16,34.61 57.16,21.27 57.8,20.64 60.02,20.64 | 60.02,20.64 BTN14.1
BTN15
  Top 0.406: R99.2 96.51,19.71 BTN15.1 93.65,20.98 92.72,21.91 92.72,28.57 92.09,29.21 67.96,29.21 66.69,30.48 66.69,34.61 68.3,36.22 IC1.7
  Bottom 0.406: BTN15.1
BTN16
  Top 0.406: BTN16.1 132.08,19.71 R112.2 136.45,19.48 136.45,19.33 136.76,19.64 138.67,19.64 139.62,20.6 139.62,34.25 133.91,39.97 76.33,39.97 IC1.13
BTN_SERIAL  (via drill 0.8 pad 1.8)
  Top 0.406: 71.04,41.23 IC1.3 72.7,41.3 73.66,42.27 v73.66,49.56 | IC2.11 76.23,106.05 74.31,106.05 73.67,105.41 v73.67,100.35
  Bottom 0.406: v73.67,100.35 v73.67,49.57 v73.66,49.56
BUTTONS  (via drill 0.8 pad 1.8)
  Top 0.406: U1.14 73.82,135.5 73.82,133.54 v73.34,132.74 | IC2.3 72.75,109.88 73.67,110.81 73.66,110.82 v73.66,115.92
  Bottom 0.406: v73.66,115.92 73.67,115.25 73.67,131.8 73.66,132.43 v73.34,132.74
GND  (via drill 0.8 pad 1.8)
  Top 0.406: 126.37,130.63 LED4.6 | U1.6 75.56,141.31 76.37,142.12 U1.29 84.78,142.12 85.01,141.88
  Bottom 0.406: v22.87,143.51 22.86,143.52 J2.3
  other vias: 70.5,100.33 69.23,32.38
  pour Bottom (isolate 1.27): 13.02,155.6 13.02,149.57 0,149.57 0,0.03 147.32,0.03 147.32,149.57 133.03,149.57 133.03,155.6
  pour Top (isolate 0.61): 13.02,155.6 13.02,149.57 0.01,149.57 0.01,0 147.32,0.03 147.32,149.57 133.03,149.57 133.03,155.6
LED_CLCK
  Top 0.406: LED1.5 21.31,132.43 21.6,132.72 21.6,137.48 23.61,139.48 65.13,139.48 66.5,138.12 U1.10
LED_DATA
  Top 0.406: U1.9 67.47,138.91 65.1,141.29 23.19,141.29 19.91,138 LED1.4
MCLR  (via drill 0.8 pad 1.8)
  Top 0.406: U1.18 77,130.96 75.26,129.22 70.81,129.22 64.22,135.81 25.81,135.81 v24.78,136.84
  Bottom 0.406: J2.1 17.78,142.56 | 17.78,142.56 17.78,142.25 | v24.78,136.84 20.65,136.84 17.79,139.7 R2.2 17.78,142.56
N$1
  Top 0.406: LED1.3 LED2.4
N$2
  Top 0.406: LED2.3 64.02,134.12 69.85,128.3 79.06,128.3 84.77,134.01 90.6,134.01 LED3.4
N$3
  Top 0.406: LED3.3 LED4.4
N$4
  Top 0.406: LED5.3 LED6.4
N$5
  Top 0.406: 84.77,149.82 C3.2 79.27,150.06 77.8,148.59 U1.37
N$6
  Top 0.406: LED6.3 63.69,98.56 65.73,96.52 86.69,96.52 88.73,98.56 LED7.4
N$7
  Top 0.406: LED8.4 LED7.3
N$8
  Top 0.406: LED9.3 LED10.4
N$9
  Top 0.406: LED10.3 LED11.4
N$10
  Top 0.406: LED11.3 LED12.4
N$11
  Top 0.406: LED13.3 LED14.4
N$12
  Top 0.406: LED14.3 LED15.4
N$13
  Top 0.406: LED16.4 LED15.3
N$14
  Top 0.406: LED8.3 140.54,98.56 143.83,95.28 143.83,71.15 142.24,69.56 17.78,69.56 15.56,67.34 15.56,63.53 16.83,62.26 19.48,62.26 LED9.4
N$15
  Top 0.406: LED12.3 140.54,62.37 143.83,59.08 143.83,15.27 134.3,5.74 17.78,5.74 12.07,11.46 12.07,23.52 15.35,26.81 LED13.4
N$16
  Top 0.406: LED1.2 LED2.5
N$17
  Top 0.406: LED2.2 63.82,132.43 69.22,127.03 80.33,127.03 85.73,132.43 LED3.5
N$18
  Top 0.406: LED3.2 LED4.5
N$19
  Top 0.406: LED4.3 140.52,134.12 141.94,132.72 141.94,120.65 139.08,117.79 21.29,117.79 19.91,116.42 LED5.4
N$20
  Top 0.406: LED4.2 139.38,132.43 140.35,131.46 140.35,121.92 137.81,119.38 19.7,119.38 16.83,116.51 16.83,97.5 17.46,96.86 LED5.5
N$21
  Top 0.406: LED6.5 LED5.2
N$22
  Top 0.406: LED6.2 63.48,96.86 64.78,95.57 87.64,95.57 88.94,96.86 LED7.5
N$23
  Top 0.406: LED8.5 LED7.2
N$24
  Top 0.406: LED8.2 140.33,96.86 142.56,94.64 142.56,71.78 141.61,70.83 17.46,70.83 14.29,67.66 14.29,63.21 16.83,60.67 LED9.5
N$25
  Top 0.406: LED9.2 LED10.5
N$26
  Top 0.406: LED10.2 LED11.5
N$27
  Top 0.406: LED11.2 LED12.5
N$28
  Top 0.406: LED12.2 140.33,60.67 142.56,58.45 142.56,16.86 133.35,7.65 18.41,7.65 13.65,12.41 13.65,22.89 15.88,25.11 LED13.5
N$29  (via drill 0.8 pad 1.8)
  other vias: 4.71,145.16
N$30
  Top 0.406: LED14.5 LED13.2
N$31
  Top 0.406: LED15.5 LED14.2
N$32
  Top 0.406: LED15.2 LED16.5
N$33  (via drill 0.8 pad 1.8)
  other vias: 4.01,4
N$34  (via drill 0.8 pad 1.8)
  other vias: 143.46,4
N$35  (via drill 0.8 pad 1.8)
  other vias: 142.73,145.17
OSC1  (via drill 0.8 pad 1.8)
  Top 0.406: U1.30 85.39,142.91 v89.85,142.9 89.78,142.98 C4.2
  Bottom 0.406: Q1.1 92.06,145.11 v89.85,142.9
OSC2  (via drill 0.8 pad 1.8)
  Top 0.406: U1.31 85.27,143.72 v86.36,144.81 87.87,146.32 C5.2
  Bottom 0.406: Q1.2 91.74,150.19 v86.36,144.81
PGC  (via drill 0.8 pad 1.8)
  Top 0.406: 75.49,135.43 U1.16 75.4,131.9 74.62,131.13 72.09,131.13 70.09,133.12 v70.09,135.22
  Bottom 0.406: J2.5 27.97,147 58.3,147 v70.09,135.22
PGD  (via drill 0.8 pad 1.8)
  Top 0.406: U1.17 76.2,131.48 74.85,130.13 71.68,130.13 64.06,137.75 v58.34,137.75
  Bottom 0.406: J2.4 25.4,140.36 28.01,137.75 v58.34,137.75
SB1  (via drill 0.8 pad 1.8)
  Top 0.406: v104.38,139.34 103.15,138.12 U1.24
  Bottom 0.406: J4.3 106.68,141.64 v104.38,139.34
SB2  (via drill 0.8 pad 1.8)
  Top 0.406: U1.23 109.67,137.31 v111.44,139.09
  Bottom 0.406: v111.44,139.09 111.44,149.74 110.41,150.77 107.24,150.77 106.68,150.22 J4.4
SB3  (via drill 0.8 pad 1.8)
  Top 0.406: U1.25 100.15,138.91 v101.28,140.04
  Bottom 0.406: J4.1 104.14,142.9 v101.28,140.04
SB4  (via drill 0.8 pad 1.8)
  Top 0.406: U1.26 97.78,139.72 v99.06,141
  Bottom 0.406: v99.06,141 100.98,142.91 100.98,147.32 101.96,148.3 J4.2
USB_D+  (via drill 0.8 pad 1.8)
  Top 0.406: U1.43 73,148.5 70.41,151.09 70.23,151.09 v70.17,151.16
  Bottom 0.406: J1.3 124.12,151.14 124.14,151.16 123.19,152.11 120.33,152.11 118.36,150.14 113.9,150.14 111.05,153 71.19,153 70.17,151.97 v70.17,151.16
USB_D-  (via drill 0.8 pad 1.8)
  Top 0.406: v124.14,143.85 119.38,143.85 110.87,152.36 73.26,152.36 72.63,151.72 72.63,150.14 73.8,148.97 U1.42
  Bottom 0.406: J1.2 124.12,143.88 v124.14,143.85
